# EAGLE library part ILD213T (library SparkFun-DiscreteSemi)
Dual Channel Phototransistor Optocoupler Dual Channel 70 V 4000 Vrms Phototransistor Optocoupler in a standard SOIC-8 package. Used to couple signals between electrically isolated circuits.
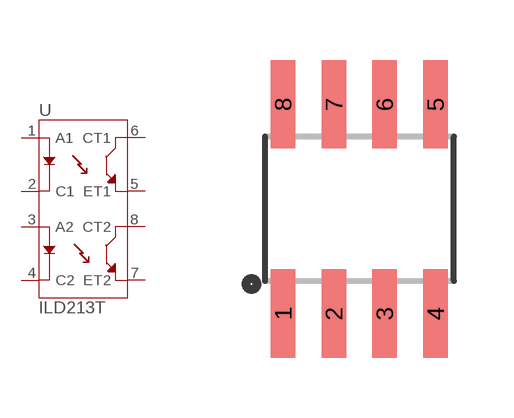
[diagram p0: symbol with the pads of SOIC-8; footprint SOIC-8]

Designator prefix U

## ILD213T (PROD_ID: IC-09076)  [SOIC-8]
1  A1
2  C1
3  A2
4  C2
5  ET1
6  CT1
7  ET2
8  CT2

## Footprint SOIC-8 (pad centres in mm)
Small Outline Package Fits JEDEC packages (narrow SOIC-8)
smd 0.61 x 2.21: 1 -1.905,-2.616; 2 -0.635,-2.616; 3 0.635,-2.616; 4 1.905,-2.616; 5 1.905,2.616; 6 0.635,2.616; 7 -0.635,2.616; 8 -1.905,2.616

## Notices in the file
Licensing: Creative Commons ShareAlike 4.0 International - https://creativecommons.org/licenses/by-sa/4.0
